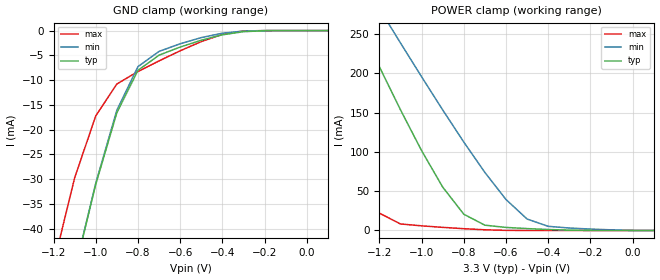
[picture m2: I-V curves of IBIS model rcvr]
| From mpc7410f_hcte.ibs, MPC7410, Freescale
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| *   rcvr  Model   *
[Model]   rcvr
Model_type   Input
Polarity   Non-Inverting
Vinl =   0.8V
Vinh =   2V
|   typ   min   max
C_comp   2.025950e-12   1.694500e-12   2.144000e-12
|   typ   min   max
[Voltage range]   3.3V   3.0V   3.6V
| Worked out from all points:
|   GND clamp passes 1 mA (typ) near -0.41 V on its own axis
|   POWER clamp passes 1 mA (typ) near -0.37 V on its own axis
|   Voltage(V)   I(typ)   I(min)   I(max)
[GND_clamp]
-3.3V     -573.6mA   -573.6mA   -554.5mA
-1.2V     -68.14mA   -68.09mA   -47.21mA
-1.1V     -48.65mA   -48.53mA   -29.75mA
-1V       -31.06mA   -30.82mA   -17.23mA
-900mV    -16.59mA   -16.09mA   -10.79mA
-800mV    -8.03mA    -7.275mA   -8.27mA
-700mV    -4.962mA   -4.205mA   -6.122mA
-600mV    -3.326mA   -2.662mA   -4.082mA
-500mV    -1.945mA   -1.418mA   -2.226mA
-400mV    -852.6uA   -526.2uA   -766.5uA
-300mV    -219.8uA   -102.6uA   -83.89uA
100mV     0A         0A         0A
[POWER_clamp]
-3.3V     1.47A      1.232A     1.706A
-1.6V     439.8mA    459.7mA    294.4mA
-1.5V     380.8mA    415mA      216.3mA
-1.3V     264.8mA    326.2mA    72.71mA
-1.2V     208.3mA    282.2mA    22.1mA
-1.1V     153.6mA    238.6mA    8.287mA
-900mV    55.25mA    153.4mA    3.975mA
-800mV    20.69mA    112.5mA    2.251mA
-700mV    6.731mA    73.82mA    874.4uA
-500mV    2.403mA    14.54mA    5.736uA
-400mV    1.212mA    5.276mA    0A
100mV     0A         0A         0A
